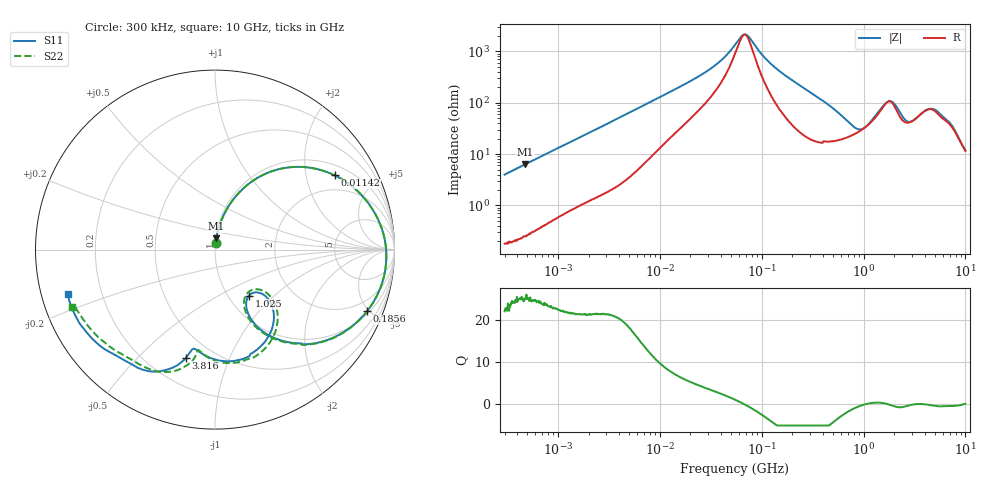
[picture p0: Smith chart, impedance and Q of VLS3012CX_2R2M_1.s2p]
! S-Parameter Data Generated by TDK Corporation
! Copyright(C) 2019 TDK Corporation.
! All Rights Reserved.
! TDK P/N: VLS3012CX-2R2M-1 (Inductor)
! Property: L=2.2uH at 1MHz
! Size(LxWxT): 3x3x1.2mm
! Model Type: s2p (Touchstone File Format Version 1.0)
! Frequency: DC=Yes Start=0.3MHz Stop=10000MHz 802points Log-sweep
! Model Generated on Sep. 23, 2019
! Port Assignments:
!  1 ---@@@--- 2
! Applicable Conditions:
!  Temperature = 25 degC
!  DC Bias Current = 0 A
!  Small Signal Operation
! Terms and conditions regarding TDK Simulation Models
! (1)This simulation model is being provided solely for informational purposes. Please refer to the specifications of the products in terms of detailed characteristics of such products.
! (2)In no event shall TDK Corporation of any of its subsidiaries be liable for any loss or damage arising, directly or indirectly,
!  From any information contained in this simulation model, including, but not limited to loss or damages arising from any inaccuracies, omissions or errors in connection with such information.
! (3)Any and all copyrights on this simulation model are owned by TDK Corporation.
!  Duplication or redistribution of this simulation model without prior written permission from TDK Corporation is prohibited.
! (4)This simulation model is subject to any modification or change without any prior notice.
! (5)Neither TDK Corporation nor any of its subsidiaries shall make any warranty, express or implied,
!  Including but not limited to the correctness, implied warranties of merchantability and fitness for a particular purpose with respect to this simulation models.
! (6)The use of this simulation model shall be deemed to have consented to the terms and conditions hereof.
# Hz S MA R 50
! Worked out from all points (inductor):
!   801 points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, 300 kHz to 10 GHz, reference 50 ohm
!   read as one part in series: L = 2.11 uH near 318.3 kHz
!   highest Q = 25.1 at 478.9 kHz (marker M1), where L = 2.11 uH
!   self-resonance near 67.92 MHz
!   S11 on the Smith chart (normalised r, x): 300 kHz: 1.00, +0.08; 11.42 MHz: 1.36, +2.93; 185.6 MHz: 1.17, -4.86; 1.025 GHz: 1.24, -0.71; 3.816 GHz: 0.36, -0.70; 10 GHz: 0.08, -0.15
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300000  0.03953 85.0  0.9974 -2.3  0.9974 -2.3  0.0394 85.2
478871  0.06281 84.1  0.9955 -3.6  0.9955 -3.6  0.06276 84.1
1713600  0.2131 75.0  0.9671 -12.3  0.967 -12.3  0.2131 75.0
3822232  0.4285 61.8  0.8829 -25.4  0.883 -25.4  0.4284 61.8
9671944  0.7426 36.4  0.6003 -47.9  0.6003 -47.9  0.7426 36.4
1.141897e7  0.7845 31.9  0.536 -51.5  0.5359 -51.5  0.7845 31.8
3.075078e7  0.923 10.7  0.2082 -63.5  0.2083 -63.5  0.923 10.7
5.477226e7  0.951 1.5  0.07102 -46.4  0.07103 -46.4  0.951 1.5
7.160072e7  0.9557 -2.7  0.04612 13.8  0.04613 13.8  0.9557 -2.7
1.063884e8  0.9526 -9.6  0.1239 61.3  0.1239 61.3  0.9525 -9.6
1.855783e8  0.9139 -22.1  0.2977 59.8  0.2977 59.8  0.9137 -22.3
3.126428e8  0.8063 -38.5  0.5045 44.6  0.5045 44.6  0.806 -38.8
6.407886e8  0.4896 -61.3  0.7332 10.5  0.7332 10.5  0.4859 -62.2
1.024756e9  0.3191 -53.6  0.7276 -16.9  0.7275 -16.9  0.3037 -54.2
1.371335e9  0.3972 -42.8  0.6019 -34.8  0.6017 -34.8  0.3824 -40.0
1.767019e9  0.5671 -58.2  0.4243 -36.1  0.4244 -36.1  0.5808 -55.8
2.08171e9  0.6285 -75.4  0.4384 -26.7  0.4386 -26.7  0.6401 -76.7
2.53795e9  0.6 -93.5  0.5269 -34.8  0.5271 -34.7  0.5982 -94.5
3.135132e9  0.5647 -102.0  0.5063 -53.1  0.5065 -53.1  0.5683 -99.7
3.816223e9  0.6244 -105.0  0.4015 -66.2  0.4017 -66.2  0.6278 -101.3
5.930102e9  0.7898 -125.9  0.2924 -68.7  0.2925 -68.8  0.7667 -124.6
1e10  0.8574 -163.2  0.2359 -90.9  0.2356 -90.9  0.8573 -158.1
